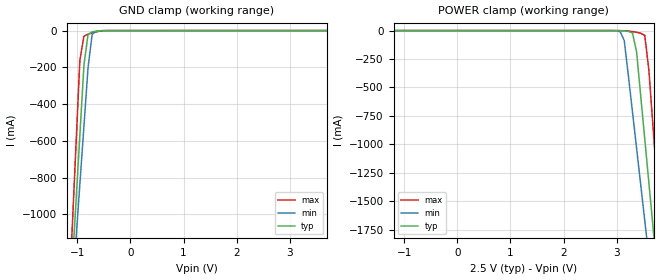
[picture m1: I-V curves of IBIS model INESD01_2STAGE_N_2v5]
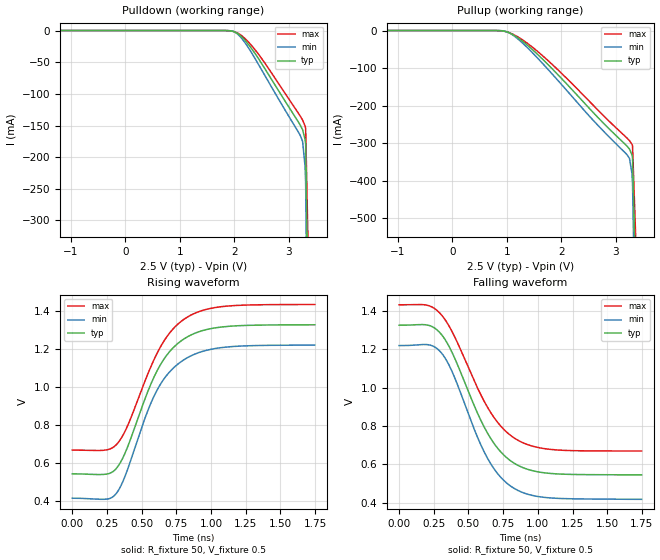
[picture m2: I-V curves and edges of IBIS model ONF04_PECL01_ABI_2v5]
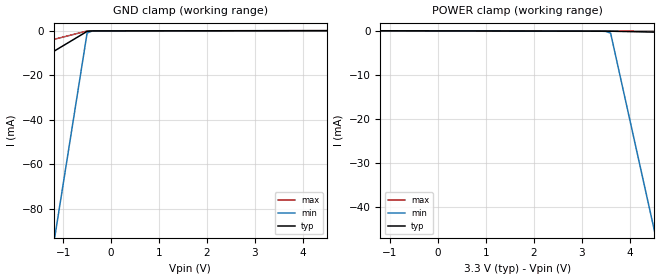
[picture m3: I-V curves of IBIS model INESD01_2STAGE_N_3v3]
|   This file is an IBIS representation of the   |
|   Integrated Device Technology , Inc.   |
|   ICS843001CI   |
|   FEMTOCLOCK CRYSTAL-TO-3.3V, 2.5V LVPECL CLOCK GENERATOR   |
[IBIS Ver]   4.1
[File name]   843001ci.ibs
[File Rev]   1.0
[Date]   27 Oct 2009 | Last modified
[Source]   Originated at Integrated Device Technology, Inc.
[Disclaimer]
IDT hereby grants the user of this IBIS model a non-exclusive,
nontransferable license to use this IBIS model under the following terms.
Before using this IBIS model, the user should read this license.
If the user does not accept these terms,  the IBIS model should be
returned to IDT within 30 days.
   The user is granted this license only to use the IBIS model and
is not granted rights to sell, load, rent, lease or license the IBIS
model in whole or in part, or in modified form to anyone other than
user. User may modify the IBIS model to suit its specific
applications but rights to derivative works and such modifications
shall belong to IDT.
   This IBIS model is provided on an "AS IS" basis and IDT makes
absolutely no warranty with respect to the information contained
herein. IDT DISCLAIMS AND CUSTOMER WAIVES ALL WARRANTIES, EXPRESS
OR IMPLIED, INCLUDING WARRANTIES OF MERCHANTABILITY OR FITNESS FOR
A PARTICULAR PURPOSE. The entire risk as to quality and performance
is with the Customer. ACCORDINGLY, IN NO EVENT SHALL THE COMPANY BE
LIABLE FOR ANY DAMAGES, WHETHER IN CONTRACT OR TORT,INCLUDING ANY
LOST PROFITS OR OTHER INCIDENTAL, CONSEQUENTIAL, EXEMPLARY, OR
PUNITIVE DAMAGES ARISING OUT OF THE USE OR APPLICATION OF THE IBIS
model provided in this package. Further, IDT reserves the right to
make changes without notice to any product herein to improve
reliability, function, or design. IDT does not convey any license
under patent rights or any other intellectual property rights,
including those of third parties.
   IDT is not obligated to provide maintenance or support
for the licensed IBIS model.
[Copyright]   Copyright 2004 by Integrated Device Technology , Inc.
[Component]   ICS843001CI
[Manufacturer] Integrated Device Technology, Inc.
[Package]
|TSSOP 8 Lead
|   typ   min   max
R_pkg   52.5m   48.8m   56.2m
L_pkg   1.381nH   1.275nH   1.486nH
C_pkg   0.236pF   0.230pF   0.242pF
[Pin]  signal_name  model_name   R_pin   L_pin   C_pin
1   VCCA   POWER   56.2m   1.486n   0.242p
2   VEE   GND   48.8m   1.275n   0.230p
3   XTAL_OUT   nc   48.8m   1.275n   0.230p
4   XTAL_IN   nc   56.2m   1.468n   0.242p
5   FREQ_SEL   INESD01_2STAGE_N   56.2m   1.486n   0.242p
6   nQ0   ONF04_PECL01_ABI   48.8m   1.275n   0.230p
7   Q0   ONF04_PECL01_ABI   48.8m   1.275n   0.230p
8   VCC   POWER   56.2m   1.468n   0.242p
[Diff Pin]  inv_pin  vdiff tdelay_typ tdelay_min  tdelay_max
7   6   NA   0  0  0
[Model Selector] INESD01_2STAGE_N
INESD01_2STAGE_N_2v5  Buffer selection for 2v5
INESD01_2STAGE_N_3v3  Buffer selection for 3v3
[Model Selector] ONF04_PECL01_ABI
ONF04_PECL01_ABI_2v5  Buffer selection for 2v5
ONF04_PECL01_ABI_3v3  Buffer selection for 3v3
| Models and submodels in the file (4): INESD01_2STAGE_N_2v5 (Input), ONF04_PECL01_ABI_2v5 (Output_ECL), INESD01_2STAGE_N_3v3 (Input), ONF04_PECL01_ABI_3v3 (Output_ECL)
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[Model] INESD01_2STAGE_N_2v5
Model_type   Input
Polarity   Non-Inverting
Vinl = .8V
Vinh = 2V
|   typ   min   max
C_comp   2pF   1.5pF   2.5pF
|   typ   min   max
[Voltage range]  2.5V   2.375V   2.625V
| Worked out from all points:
|   GND clamp passes 1 mA (typ) near -0.56 V on its own axis
[GND_clamp]
|Voltage   I(typ)   I(min)   I(max)
-2.5V     -8.269A    -7.245A    -9.986A
-1.108V   -1.338A    -1.475A    -1.143A
-1.031V   -954.2mA   -1.155A    -652.3mA
-953.6mV  -570.3mA   -836.3mA   -161.2mA
-876.3mV  -186.9mA   -517.7mA   -30.19mA
-799mV    -20.06mA   -199.8mA   -19.86mA
-721.6mV  -7.024mA   -20.98mA   -12.73mA
-644.3mV  -3.118mA   -2.836mA   -6.727mA
-489.7mV  -245.9uA   -116.3uA   -585.7uA
5V        96.94uA    121.2uA    75.12uA
[POWER_clamp]
|Voltage   I(typ)   I(min)   I(max)
-2.5V     96.94uA    118.2uA    76.99uA
3.067V    -1.047mA   -9.228mA   -195uA
3.144V    -3.118mA   -87.68mA   -1.083mA
3.299V    -20.06mA   -714.1mA   -8.863mA
3.376V    -186.9mA   -1.033A    -15.35mA
3.454V    -570.3mA   -1.352A    -22.94mA
3.531V    -954.2mA   -1.672A    -42.29mA
3.608V    -1.338A    -1.991A    -349.4mA
3.686V    -1.723A    -2.311A    -840.5mA
3.763V    -2.108A    -2.632A    -1.332A
3.84V     -2.492A    -2.952A    -1.823A
5V        -8.269A    -7.765A    -9.192A
[Model] ONF04_PECL01_ABI_2v5
Model_type   Output_ECL
Polarity   Non-Inverting
|   typ   min   max
C_comp   2pF   1.5pF   2.5pF
Vmeas = 0.930V
Rref = 50
Cref = 0
Vref = 0.5V
|   typ   min   max
[Voltage range]   2.5V   2.375V   2.625V
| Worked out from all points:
|   rising waveform, R_fixture 50, V_fixture 0.5: 20-80 % time 277ps typ, 275ps min, 285ps max; typ from 0.545 V to 1.32 V
|   falling waveform, R_fixture 50, V_fixture 0.5: 20-80 % time 301ps typ, 287ps min, 316ps max; typ from 1.32 V to 0.545 V
[Pulldown]
|Voltage   I (typ)   I (min)   I (max)
-2.5V     6.875pA    6.75pA     8.541pA
1.832V    -49.43uA   -26.45uA   -64.94uA
1.97V     -1.182mA   -1.109mA   -1.119mA
2.062V    -4.795mA   -5.652mA   -4.061mA
2.245V    -20.49mA   -25.42mA   -16.92mA
2.474V    -48.52mA   -58.16mA   -40.96mA
3.208V    -149mA     -165.2mA   -134.7mA
3.254V    -156.7mA   -175mA     -141.4mA
3.3V      -172.3mA   -215.3mA   -150.9mA
3.31V     -179.1mA   -241mA     -154mA
3.648V    -2.077A    -2.874A    -1.569A
5V        -10.5A     -13.61A    -8.602A
[Pullup]
|Voltage   I (typ)   I (min)   I (max)
-2.5V     6.875pA    6.75pA     8.541pA
869.3mV   -314.1uA   -153uA     -446.4uA
1.007V    -3.871mA   -3.675mA   -3.835mA
1.099V    -9.86mA    -10.92mA   -8.943mA
1.374V    -38.48mA   -44.94mA   -33.5mA
1.741V    -88.13mA   -100.7mA   -77.72mA
2.52V     -207.7mA   -228.2mA   -188.7mA
3.254V    -315.2mA   -340mA     -292.9mA
3.3V      -330.9mA   -380.3mA   -302.6mA
3.31V     -337.7mA   -406.1mA   -305.8mA
3.648V    -2.236A    -3.039A    -1.722A
5V        -10.66A    -13.77A    -8.757A
[Ramp]
|   typ   min   max
dV/dt_r   0.627/0.437n   0.646/0.439n   0.611/0.444n
dV/dt_f   0.626/0.462n   0.645/0.442n   0.611/0.484n
R_load =   50.0000
[Rising Waveform]
R_fixture = 50
V_fixture = 0.5   | VCC_typ - 2V
V_fixture_max = 0.625   | VCC_max - 2V
V_fixture_min = 0.375   | VCC_min - 2V
C_fixture = 0.0p
| Time   typ   min   max
0s        544.6mV    417.1mV    669mV
247ps     543.4mV    412.2mV    670.1mV
315.3ps   571.2mV    440.4mV    695.7mV
397.6ps   683.4mV    565.4mV    794.5mV
523.8ps   936.8mV    835.4mV    1.03V
600.9ps   1.069V     968.4mV    1.161V
697.2ps   1.181V     1.075V     1.278V
805.8ps   1.251V     1.142V     1.354V
1.083ns   1.314V     1.206V     1.421V
1.748ns   1.325V     1.219V     1.431V
[Falling Waveform]
R_fixture = 50
V_fixture = 0.5   | VCC_typ - 2V
V_fixture_max = 0.625   | VCC_max - 2V
V_fixture_min = 0.375   | VCC_min - 2V
C_fixture = 0.0p
| Time   typ   min   max
0s        1.325V     1.219V     1.432V
208.5ps   1.325V     1.224V     1.428V
308.3ps   1.274V     1.178V     1.376V
387.1ps   1.175V     1.074V     1.284V
550ps     891.1mV    767.3mV    1.021V
627.1ps   775.5mV    645mV      910.1mV
718.2ps   676.7mV    544.2mV    811.3mV
819.8ps   610.1mV    478.6mV    742mV
1.086ns   552.7mV    425mV      678.1mV
1.748ns   545mV      417.5mV    669.3mV
[Model] INESD01_2STAGE_N_3v3
Model_type   Input
Polarity   Non-Inverting
Vinl = 0.8V
Vinh = 2.0V
|   typ   min   max
C_comp   2pF   1.5pF   2.5pF
|   typ   min   max
[Voltage range]  3.3V   3.15V   3.45V
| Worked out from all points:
|   GND clamp passes 1 mA (typ) near -0.56 V on its own axis
[GND_clamp]
|Voltage   I(typ)   I(min)   I(max)
-3.3V     -36.4mA    -382.1mA   -15.22mA
-1.2V     -9.271mA   -96.28mA   -3.853mA
-1.1V     -7.979mA   -82.66mA   -3.312mA
-500mV    -227.8uA   -989.9uA   -65.11uA
-400mV    -30.81uA   -105.6uA   -11.01uA
-300mV    -7.585uA   -16.23uA   -6.189uA
6.6V      129.3uA    124.7uA    134.2uA
[POWER_clamp]
|Voltage   I(typ)   I(min)   I(max)
-3.3V     129.3uA    121.5uA    137.6uA
3.4V      -1.963uA   -9.687uA   1.322uA
3.5V      -4.012uA   -52.24uA   -711.7nA
3.6V      -7.585uA   -433.5uA   -2.745uA
4.5V      -216.6uA   -44.85mA   -21.11uA
4.6V      -239.9uA   -49.78mA   -23.15uA
6.6V      -704.4uA   -148.5mA   -63.97uA
